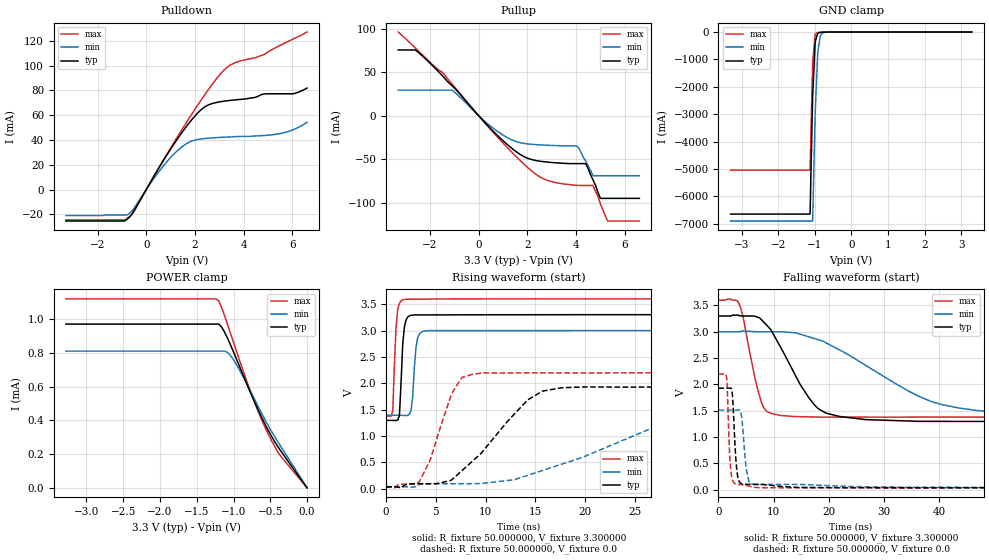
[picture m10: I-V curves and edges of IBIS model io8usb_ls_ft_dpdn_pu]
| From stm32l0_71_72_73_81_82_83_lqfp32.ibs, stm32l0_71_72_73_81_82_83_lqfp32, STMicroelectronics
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|   Model io8usb_ls_ft_dpdn_pu
[Model]  io8usb_ls_ft_dpdn_pu
Model_type I/O
Polarity   Non-Inverting
Enable   Active-Low
Vinl =   0.990000V
Vinh =   2.310000V
Vmeas =  1.650000V
Cref =   50.000000pF
Rref =   100.000000M
Vref =   0.0V
C_comp   4.637700pF   4.584200pF   4.727200pF
[Temperature Range]   25.000000   0.125000k   -40.000000
[Pullup Reference]   3.300000V   3.000000V   3.600000V
[Pulldown Reference]   0.0V   0.0V   0.0V
[POWER Clamp Reference]   3.300000V   3.000000V   3.600000V
[GND Clamp Reference]   0.0V   0.0V   0.0V
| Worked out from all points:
|   slope of the pulldown table from 0 to 0.495 V, typ, clamps not added: 29.7 ohm
|   slope of the pullup table from 0 to 0.495 V, typ, clamps not added: 33.1 ohm
|   GND clamp passes 1 mA (typ) near -0.59 V on its own axis
|   rising waveform, R_fixture 50.000000, V_fixture 3.300000: 20-80 % time 333ps typ, 350ps min, 312ps max; typ from 1.3 V to 3.3 V
|   rising waveform, R_fixture 50.000000, V_fixture 0.0: 20-80 % time 5.52ns typ, 12.4ns min, 2.29ns max; typ from 0.036 V to 1.93 V
|   falling waveform, R_fixture 50.000000, V_fixture 3.300000: 20-80 % time 6.51ns typ, 16.2ns min, 2.63ns max; typ from 3.3 V to 1.3 V
|   falling waveform, R_fixture 50.000000, V_fixture 0.0: 20-80 % time 605ps typ, 788ps min, 503ps max; typ from 1.93 V to 0.036 V
[Pulldown]
|Voltage   I(typ)   I(min)   I(max)
-3.3V     -25.4mA    -21mA      -24.51mA
-900mV    -25.4mA    -20.55mA   -24.51mA
-700mV    -22.51mA   -19.36mA   -21.96mA
500mV     16.83mA    13.94mA    16.94mA
1.2V      38.51mA    29.82mA    39.91mA
1.8V      54.63mA    38.53mA    58.7mA
2.4V      66.61mA    41.1mA     76.36mA
3.4V      71.77mA    42.37mA    99.7mA
4.8V      76.87mA    43.51mA    108.6mA
5.5V      77.19mA    45.13mA    116.3mA
6.1V      77.54mA    48.75mA    122mA
6.6V      81.82mA    54.26mA    127mA
[Pullup]
|Voltage   I(typ)   I(min)   I(max)
-3.3V     75.42mA    29.26mA    95.99mA
-2.6V     75.42mA    29.26mA    77.76mA
-1.1V     34.75mA    29.26mA    36.77mA
900mV     -26.17mA   -20.49mA   -28.4mA
2.3V      -51.24mA   -33.18mA   -66.19mA
2.9V      -53.55mA   -34.11mA   -75.01mA
4V        -55.1mA    -34.59mA   -79.98mA
4.4V      -55.1mA    -52mA      -80.17mA
4.7V      -74mA      -69mA      -80.17mA
5V        -95mA      -69mA      -101mA
5.3V      -95mA      -69mA      -121mA
6.6V      -95mA      -69mA      -121mA
[GND_clamp]
|Voltage   I(typ)   I(min)   I(max)
-3.3V     -6.648A    -6.902A    -5.041A
-1.13V    -6.648A    -6.902A    -5.041A
-1.06V    -2.348A    -6.902A    -1.115A
-990mV    -354.4mA   -2.925A    -78.01mA
-920mV    -39.6mA    -752.9mA   -17.76mA
-850mV    -11.68mA   -132.4mA   -11.58mA
-780mV    -6.831mA   -24.65mA   -7.717mA
-500mV    -137.7uA   -388.6uA   -81.08uA
3.28V     0A         0A         0A
[POWER_clamp]
|Voltage   I(typ)   I(min)   I(max)
-3.28V    971.8uA    811.6uA    1.121mA
-1.24V    971.8uA    811.6uA    1.121mA
-1.2V     971.8uA    811.6uA    1.109mA
-1.16V    953uA      811.6uA    1.068mA
-1.08V    886.6uA    802.8uA    968.1uA
-1V       806.6uA    760.2uA    863.7uA
-920mV    722.5uA    701.2uA    759.8uA
-760mV    555.9uA    565.7uA    561.9uA
-640mV    439.3uA    461.7uA    428.2uA
-560mV    368uA      395.1uA    348.6uA
-400mV    247.1uA    275.7uA    213.9uA
0V        0A         0A         0A
[Ramp]
| variable   typ   min   max
dV/dt_r  1.13573/5.52000n   0.88396/12.37278n   1.29812/2.28992n
dV/dt_f  1.20216/6.49918n   0.96414/16.13081n   1.33236/2.62781n
R_load = 50.000000
[Rising Waveform]
R_fixture= 50.000000
V_fixture= 3.300000
V_fixture_min= 3.000000
V_fixture_max= 3.600000
|time   V(typ)   V(min)   V(max)
0s        1.297V     1.393V     1.378V
667.3ps   1.297V     1.393V     1.481V
1.001ns   1.294V     1.393V     3.073V
1.335ns   1.388V     1.393V     3.517V
1.668ns   2.744V     1.392V     3.583V
1.835ns   3.068V     1.39V      3.589V
2.503ns   3.288V     1.484V     3.592V
3.17ns    3.296V     2.863V     3.593V
4.004ns   3.296V     2.994V     3.595V
83.08ns   3.3V       3V         3.6V
[Rising Waveform]
R_fixture= 50.000000
V_fixture= 0.0
V_fixture_min= 0.0
V_fixture_max= 0.0
|time   V(typ)   V(min)   V(max)
0s        36.32mV    40.23mV    34.36mV
3.337ns   96.08mV    80.23mV    134.4mV
4.505ns   95.28mV    97.58mV    586.9mV
6.673ns   181.7mV    96.83mV    1.827V
7.674ns   351.6mV    96.84mV    2.114V
8.842ns   549.8mV    97.6mV     2.175V
14.18ns   1.672V     251.2mV    2.198V
17.68ns   1.916V     468.1mV    2.197V
31.36ns   1.93V      1.428V     2.196V
83.08ns   1.928V     1.512V     2.196V
[Falling Waveform]
R_fixture= 50.000000
V_fixture= 3.300000
V_fixture_min= 3.000000
V_fixture_max= 3.600000
|time   V(typ)   V(min)   V(max)
0s        3.3V       3V         3.6V
3.837ns   3.305V     3.001V     3.504V
7.341ns   3.269V     3V         1.814V
8.175ns   3.187V     3V         1.559V
9.676ns   3.005V     3V         1.444V
17.35ns   1.614V     2.873V     1.381V
21.86ns   1.391V     2.658V     1.379V
36.2ns    1.298V     1.778V     1.379V
43.54ns   1.297V     1.551V     1.379V
83.08ns   1.297V     1.393V     1.378V
[Falling Waveform]
R_fixture= 50.000000
V_fixture= 0.0
V_fixture_min= 0.0
V_fixture_max= 0.0
|time   V(typ)   V(min)   V(max)
0s        1.928V     1.512V     2.196V
1.502ns   1.928V     1.512V     2.113V
2.002ns   1.928V     1.512V     697mV
2.336ns   1.923V     1.512V     272mV
2.669ns   1.556V     1.512V     150.2mV
3.17ns    541.2mV    1.512V     105.4mV
4.004ns   122.5mV    1.492V     96.04mV
5.005ns   99.49mV    417.3mV    81.96mV
6.173ns   98.71mV    106mV      48.08mV
83.08ns   36.32mV    40.23mV    34.36mV
